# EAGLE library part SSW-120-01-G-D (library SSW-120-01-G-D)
40 Position, .100" Tiger Buy Socket Strip Source: Datasheet
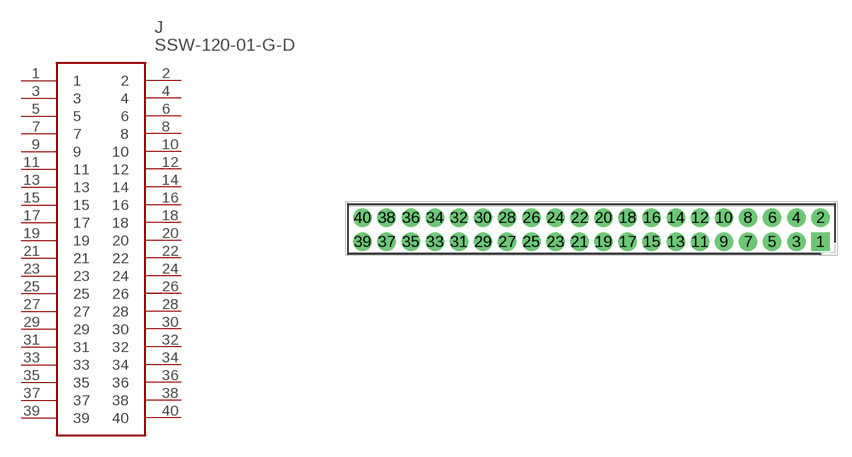
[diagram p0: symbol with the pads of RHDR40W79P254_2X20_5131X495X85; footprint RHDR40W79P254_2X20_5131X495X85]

Designator prefix J

## SSW-120-01-G-D (Description: 40 Position, .100" Tiger Buy Socket Strip; Height: 8.51mm; Manufacturer_Name: SAMTEC; Manufacturer_Part_Number: SSW-120-01-G-D; Mouser_Part_Number: 200-SSW12001GD; Mouser_Price-Stock: https://www.mouser.co.uk/ProductDetail/Samtec/SSW-120-01-G-D?qs=NxGO64s6WXgWmpEZA9sU8w%3D%3D)  [RHDR40W79P254_2X20_5131X495X85]
1  1
2  2
3  3
4  4
5  5
6  6
7  7
8  8
9  9
10  10
11  11
12  12
13  13
14  14
15  15
16  16
17  17
18  18
19  19
20  20
21  21
22  22
23  23
24  24
25  25
26  26
27  27
28  28
29  29
30  30
31  31
32  32
33  33
34  34
35  35
36  36
37  37
38  38
39  39
40  40

## Footprint RHDR40W79P254_2X20_5131X495X85 (pad centres in mm)
SSW-120-01-G-D
drill 1.3 pad 1.95 square: 1 0,0
drill 1.3 pad 1.95: 2 0,2.54; 3 -2.54,0; 4 -2.54,2.54; 5 -5.08,0; 6 -5.08,2.54; 7 -7.62,0; 8 -7.62,2.54; 9 -10.16,0; 10 -10.16,2.54; 11 -12.7,0; 12 -12.7,2.54; 13 -15.24,0; 14 -15.24,2.54; 15 -17.78,0; 16 -17.78,2.54; 17 -20.32,0; 18 -20.32,2.54; 19 -22.86,0; 20 -22.86,2.54; 21 -25.4,0; 22 -25.4,2.54; 23 -27.94,0; 24 -27.94,2.54; 25 -30.48,0; 26 -30.48,2.54; 27 -33.02,0; 28 -33.02,2.54; 29 -35.56,0; 30 -35.56,2.54; 31 -38.1,0; 32 -38.1,2.54; 33 -40.64,0; 34 -40.64,2.54; 35 -43.18,0; 36 -43.18,2.54; 37 -45.72,0; 38 -45.72,2.54; 39 -48.26,0; 40 -48.26,2.54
